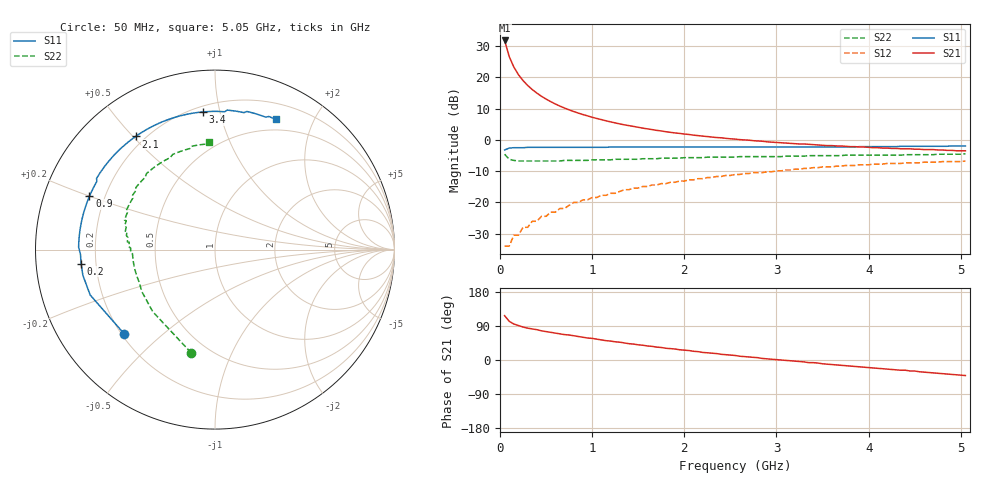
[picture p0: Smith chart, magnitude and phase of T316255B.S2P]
!AT-31625
!S-PARAMETERS at Vce=4.8 V  Ic=100 mA.  LAST UPDATED 08-05-96
# ghz s ma r 50
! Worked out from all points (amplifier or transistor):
!   101 points, 50 MHz to 5.05 GHz, reference 50 ohm
!   highest |S21| = 31.8 dB at 50 MHz (marker M1)
!   |S21| within 3 dB of that: start of sweep to 79.14 MHz
!   unconditionally stable (mu >= 1): 481.4 MHz to 536.3 MHz; 557.9 MHz to 1.331 GHz; 1.374 GHz to 1.433 GHz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
!   at 850 MHz: K = 1.04, MAG = 13.0 dB, |S12| = -20.0 dB
!   at 2.55 GHz: K = 0.96, MSG = 5.7 dB, |S12| = -11.1 dB
!   at 5.05 GHz: K = 0.93, MSG = 1.6 dB, |S12| = -6.7 dB
!   S11 on the Smith chart (normalised r, x): 50 MHz: 0.21, -0.38; 200 MHz: 0.14, -0.05; 900 MHz: 0.14, +0.20; 2.1 GHz: 0.16, +0.51; 3.4 GHz: 0.24, +0.89; 5.05 GHz: 0.37, +1.50
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0.05  0.69 -137.0  38.85 117.0  0.02 42.0  0.59 -103.0
0.1  0.74 -160.0  21.48 102.0  0.02 41.0  0.49 -135.0
0.15  0.75 -169.0  14.6 95.0  0.03 46.0  0.47 -150.0
0.2  0.75 -174.0  11.04 91.0  0.03 50.0  0.46 -157.0
0.25  0.75 -178.0  8.88 87.0  0.04 53.0  0.46 -162.0
0.3  0.76 179.0  7.42 84.0  0.04 56.0  0.46 -166.0
0.35  0.76 177.0  6.38 82.0  0.05 58.0  0.46 -168.0
0.4  0.76 174.0  5.59 80.0  0.05 60.0  0.46 -170.0
0.45  0.76 172.0  4.98 77.0  0.06 61.0  0.46 -172.0
0.55  0.76 169.0  4.09 73.0  0.07 62.0  0.46 -174.0
0.65  0.76 165.0  3.47 69.0  0.08 63.0  0.46 -177.0
0.75  0.76 162.0  3.02 66.0  0.09 63.0  0.47 -178.0
0.9  0.76 157.0  2.54 60.0  0.11 62.0  0.47 179.0
1.1  0.76 152.0  2.11 53.0  0.13 60.0  0.48 177.0
1.25  0.77 148.0  1.87 48.0  0.14 58.0  0.49 175.0
1.5  0.77 141.0  1.59 40.0  0.17 54.0  0.49 172.0
1.75  0.77 134.0  1.39 33.0  0.2 51.0  0.51 169.0
2.1  0.77 125.0  1.19 23.0  0.23 45.0  0.52 164.0
2.55  0.77 114.0  1.03 12.0  0.28 37.0  0.53 157.0
3.4  0.77 95.0  0.84 -7.0  0.36 22.0  0.56 141.0
4.25  0.78 79.0  0.73 -25.0  0.42 3.0  0.57 119.0
5.05  0.8 65.0  0.67 -41.0  0.46 -13.0  0.6 93.0
